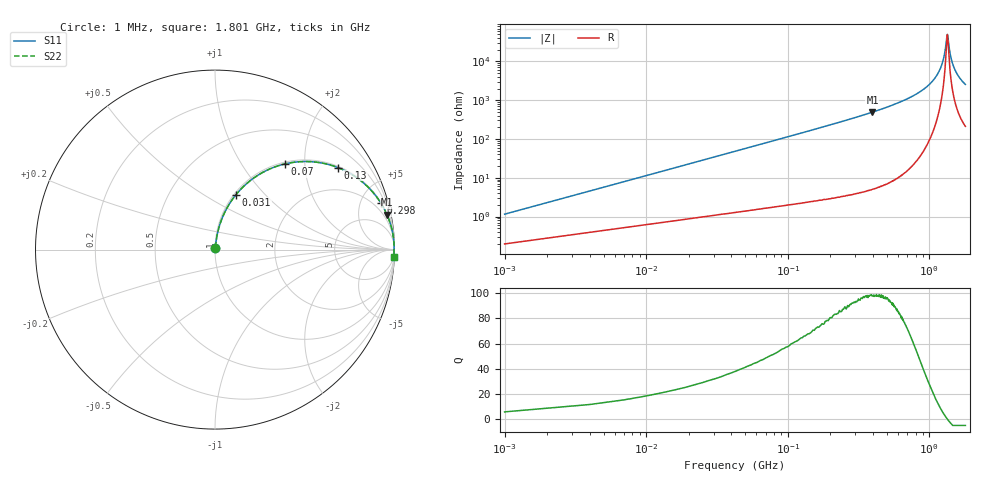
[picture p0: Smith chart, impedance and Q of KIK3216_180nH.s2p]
!version-2
!date-01.2022
!Series
# MHz S RI R 50
!Freq ReS11 ImS11 ReS21 ImS21 ReS12 ImS12 ReS22 ImS22
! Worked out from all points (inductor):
!   601 points, 1 MHz to 1.801 GHz, reference 50 ohm
!   read as one part in series: L = 180 nH near 10 MHz
!   highest Q = 98.1 at 397 MHz (marker M1), where L = 197 nH
!   self-resonance near 1.342 GHz
!   S11 on the Smith chart (normalised r, x): 1 MHz: 1.00, +0.02; 31 MHz: 1.02, +0.70; 70 MHz: 1.03, +1.59; 130 MHz: 1.05, +2.97; 298 MHz: 1.08, +7.09; 1.801 GHz: 5, -51
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1  0.00207 0.0113  0.9979 -0.0113  0.9979 -0.0113  0.00207 0.0113
13  0.0277 0.142  0.9723 -0.142  0.9723 -0.142  0.0277 0.142
16  0.0387 0.1726  0.9613 -0.1726  0.9613 -0.1726  0.0387 0.1726
31  0.1171 0.3064  0.8829 -0.3064  0.8829 -0.3064  0.1171 0.3064
70  0.3889 0.4773  0.6111 -0.4773  0.6111 -0.4773  0.3889 0.4773
130  0.6852 0.4569  0.3148 -0.4569  0.3148 -0.4569  0.6852 0.4569
199  0.8381 0.3622  0.1619 -0.3622  0.1619 -0.3622  0.8381 0.3622
298  0.9239 0.2598  0.0761 -0.2598  0.0761 -0.2598  0.9239 0.2598
301  0.9254 0.2574  0.0746 -0.2574  0.0746 -0.2574  0.9254 0.2574
397  0.9585 0.1944  0.0415 -0.1944  0.0415 -0.1944  0.9585 0.1944
601  0.985 0.1157  0.015 -0.1157  0.015 -0.1157  0.985 0.1157
901  0.9958 0.0537  0.00422 -0.0537  0.00422 -0.0537  0.9958 0.0537
1081  0.9976 0.0287  0.00235 -0.0287  0.00235 -0.0287  0.9976 0.0287
1201  0.9981 0.0147  0.00194 -0.0147  0.00194 -0.0147  0.9981 0.0147
1276  0.9981 0.00677  0.00191 -0.00677  0.00191 -0.00677  0.9981 0.00677
1342  0.998 0.000158  0.002 -0.000158  0.002 -0.000158  0.998 0.000158
1354  0.998 -0.00101  0.00203 0.00101  0.00203 0.00101  0.998 -0.00101
1387  0.9979 -0.00416  0.00212 0.00416  0.00212 0.00416  0.9979 -0.00416
1417  0.9978 -0.00697  0.00222 0.00697  0.00222 0.00697  0.9978 -0.00697
1501  0.9974 -0.0145  0.00259 0.0145  0.00259 0.0145  0.9974 -0.0145
1627  0.9966 -0.0252  0.00335 0.0252  0.00335 0.0252  0.9966 -0.0252
1801  0.9953 -0.0387  0.00474 0.0387  0.00474 0.0387  0.9953 -0.0387
